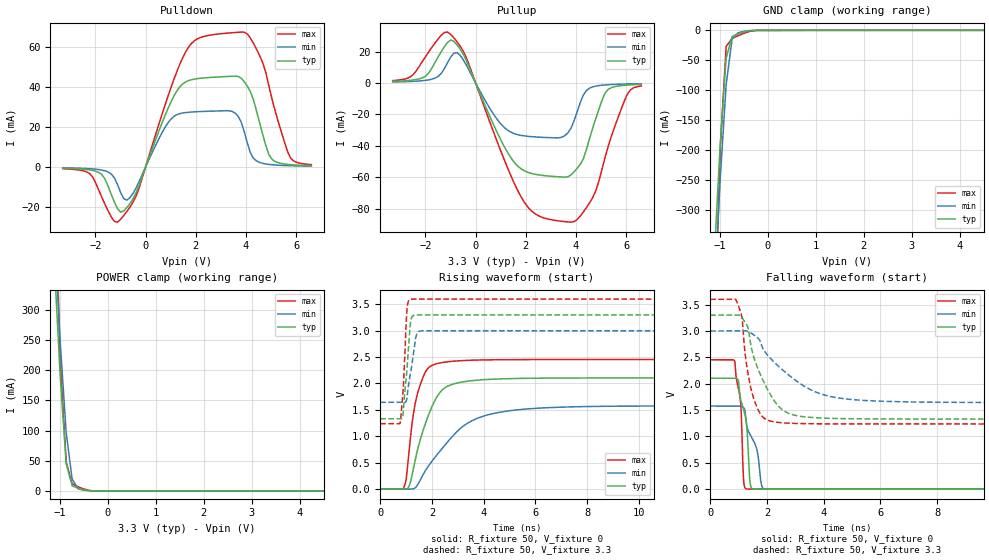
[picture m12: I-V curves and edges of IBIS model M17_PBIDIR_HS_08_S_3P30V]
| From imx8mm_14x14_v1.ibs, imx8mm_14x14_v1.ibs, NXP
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[Model] M17_PBIDIR_HS_08_S_3P30V
Model_type I/O
Vinl  =  0.99
Vinh  =  2.31
Vmeas =  1.65
| Capacitance   typ   min   max
C_comp   1.08818991111e-12   1.03117834871e-12   1.10439570077e-12
| Variables   typ   min   max
[GND Clamp Reference]   0   0   0
[POWER Clamp Reference]   3.3   3   3.6
[Pulldown Reference]   0   0   0
[Pullup Reference]   3.3   3   3.6
[Temperature Range]   25   125   -40
[Voltage Range]   3.3   3   3.6
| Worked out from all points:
|   slope of the pulldown table from 0 to 0.495 V, typ, clamps not added: 29.5 ohm
|   slope of the pullup table from 0 to 0.495 V, typ, clamps not added: 26.5 ohm
|   GND clamp passes 1 mA (typ) near -0.39 V on its own axis
|   POWER clamp passes 1 mA (typ) near -0.44 V on its own axis
|   falling waveform, R_fixture 50, V_fixture 0: 20-80 % time 285ps typ, 476ps min, 176ps max; typ from 2.11 V to 0.002 V
|   falling waveform, R_fixture 50, V_fixture 3.3: 20-80 % time 817ps typ, 1.63ns min, 393ps max; typ from 3.3 V to 1.33 V
|   rising waveform, R_fixture 50, V_fixture 0: 20-80 % time 824ps typ, 1.72ns min, 469ps max; typ from 0.002 V to 2.11 V
|   rising waveform, R_fixture 50, V_fixture 3.3: 20-80 % time 194ps typ, 249ps min, 140ps max; typ from 1.33 V to 3.3 V
[GND Clamp]
| Voltage   I(typ)   I(min)   I(max)
-3.3V     -7.236A    -6.565A    -8.004A
-1.117V   -380.4mA   -438.7mA   -546.7mA
-993.1mV  -191mA     -249.4mA   -198.9mA
-869mV    -46.61mA   -90.79mA   -26.93mA
-744.8mV  -10.31mA   -14.37mA   -13.71mA
-620.7mV  -5.945mA   -4.193mA   -9.059mA
-372.4mV  -659.7uA   -360.2uA   -1.673mA
-248.3mV  -143.8uA   -94.2uA    -265.5uA
6.6V      0A         0A         0A
[POWER Clamp]
| Voltage   I(typ)   I(min)   I(max)
-3.3V     7.237A     6.564A     8.009A
-1.117V   380.7mA    433.6mA    553.5mA
-993.1mV  190.7mA    247mA      219.9mA
-869mV    45.33mA    97.36mA    48.38mA
-744.8mV  8.677mA    19.82mA    11.82mA
-620.7mV  4.425mA    3.499mA    6.828mA
-372.4mV  215.5uA    293.3uA    764.6uA
-248.3mV  4.273uA    22.4uA     51.08uA
6.6V      0A         0A         0A
[Pulldown]
| Voltage   I(typ)   I(min)   I(max)
-3.3V     -630.6uA   -436.3uA   -874.4uA
-2.234V   -1.472mA   -870.7uA   -3.23mA
-1.738V   -3.836mA   -1.563mA   -15.22mA
-1.117V   -20.73mA   -8.828mA   -27.52mA
-620.7mV  -18.2mA    -15.24mA   -19.99mA
910.3mV   29.63mA    22.28mA    35.87mA
1.707V    42.99mA    27.23mA    59.6mA
3.797V    44.31mA    22.69mA    67.16mA
4.293V    33.61mA    4.356mA    61.66mA
5.038V    3.752mA    1.089mA    33.65mA
5.783V    1.129mA    606.5uA    4.292mA
6.6V      640.6uA    405.9uA    1.146mA
[Pullup]
| Voltage   I(typ)   I(min)   I(max)
-3.3V     968.4uA    609.2uA    1.472mA
-2.607V   1.636mA    918.8uA    3.746mA
-1.986V   4.378mA    1.647mA    16.9mA
-993.1mV  27.31mA    16.37mA    30.93mA
-620.7mV  21.69mA    17.71mA    23.62mA
1.024V    -36.96mA   -26.46mA   -44.17mA
1.934V    -55.91mA   -33.74mA   -75.84mA
3.797V    -58.63mA   -28.93mA   -88.71mA
4.417V    -42.26mA   -4.748mA   -79.32mA
5.162V    -6.292mA   -1.277mA   -47.12mA
6.031V    -1.361mA   -679.7uA   -7.568mA
6.6V      -914.7uA   -518.8uA   -1.915mA
[Ramp]
dV/dt_r   1.26224/0.823885n  0.945763/1.72345n  1.47108/0.468799n
dV/dt_f   1.18172/0.816793n  0.814588/1.63145n  1.41756/0.39282n
R_load = 50
[Falling Waveform]
R_fixture = 50
V_fixture = 0
V_fixture_min = 0
V_fixture_max = 0
| Time   V(typ)   V(min)   V(max)
0s        2.106V     1.578V     2.454V
863.7ps   2.105V     1.578V     2.422V
1.075ns   1.693V     1.576V     1.608V
1.183ns   1.498V     1.542V     120.3mV
1.284ns   1.197V     1.217V     5.75mV
1.351ns   557.6mV    1.091V     3.693mV
1.451ns   25.46mV    990.4mV    3.472mV
1.819ns   2.497mV    56.6mV     2.916mV
2.072ns   2.283mV    2.18mV     2.836mV
333.3ns   1.826mV    1.245mV    2.522mV
[Falling Waveform]
R_fixture = 50
V_fixture = 3.3
V_fixture_min = 3
V_fixture_max = 3.6
| Time   V(typ)   V(min)   V(max)
0s        3.3V       3V         3.6V
941ps     3.302V     3V         3.549V
1.122ns   3.246V     3.001V     3.243V
1.247ns   3.147V     3.005V     2.486V
1.408ns   2.803V     2.969V     1.971V
1.82ns    2.109V     2.71V      1.389V
2.521ns   1.516V     2.275V     1.26V
3.546ns   1.361V     1.884V     1.242V
11.35ns   1.33V      1.643V     1.237V
333.3ns   1.33V      1.642V     1.237V
[Rising Waveform]
R_fixture = 50
V_fixture = 0
V_fixture_min = 0
V_fixture_max = 0
| Time   V(typ)   V(min)   V(max)
0s        1.826mV    1.245mV    2.522mV
925.6ps   -1.961mV   1.188mV    43.21mV
1.006ns   582.3uV    -279uV     201.9mV
1.13ns    71.21mV    -355.7uV   793.8mV
1.348ns   542.4mV    21mV       1.616V
1.825ns   1.349V     410.1mV    2.275V
2.507ns   1.922V     836.8mV    2.405V
4.071ns   2.074V     1.393V     2.448V
13.07ns   2.106V     1.577V     2.454V
333.3ns   2.106V     1.578V     2.454V
[Rising Waveform]
R_fixture = 50
V_fixture = 3.3
V_fixture_min = 3
V_fixture_max = 3.6
| Time   V(typ)   V(min)   V(max)
0s        1.33V      1.642V     1.237V
775.1ps   1.33V      1.642V     1.264V
875.4ps   1.392V     1.642V     1.811V
998.9ps   2.069V     1.662V     3.141V
1.033ns   2.272V     1.733V     3.406V
1.146ns   3.058V     2.126V     3.593V
1.228ns   3.263V     2.373V     3.598V
1.413ns   3.298V     2.94V      3.599V
1.764ns   3.299V     2.999V     3.599V
333.3ns   3.3V       3V         3.6V
[Add Submodel]
| Submodel Name Mode
M17_PBIDIR_HS_08_S_3P30V_T All
